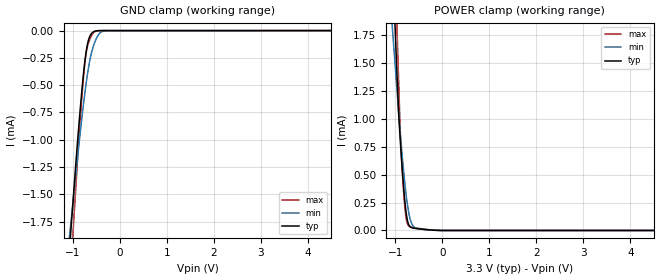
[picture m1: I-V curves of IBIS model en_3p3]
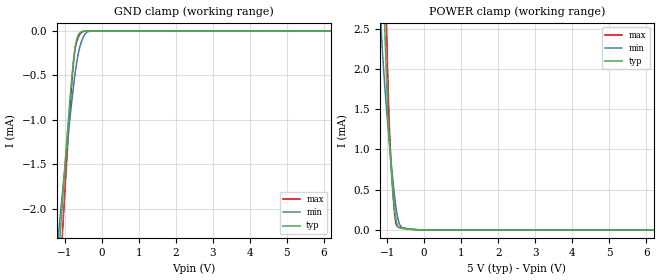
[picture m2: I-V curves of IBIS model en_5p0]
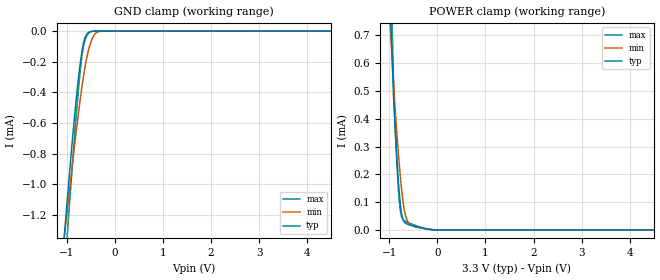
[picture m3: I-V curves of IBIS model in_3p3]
|Texas Instruments Incorporated
| ISO734x Robust EMC, Low Power, Quad-Channel Digital Isolators
| Marketing part#   Digital Voltage Range   Package-type   #pins
| ISO7341CDW   3.0V - 5.5V   SOIC   16
[IBIS Ver]   4.1
[File name]   iso7341c.ibs
[File Rev]   1.1
[Date]   9/10/2014
[Source]
| Texas Instruments Incorporated.
| Analog-eLab Design Center, HPA
| 12500 TI Blvd
| Dallas, TX -75243
[Notes]   Revision History:
| Rev 1.1: 9/10/2014
| - output_3p3 and output_5p0 modeled as tri-state buffers.
| Rev 1.0: 8/19/2014
| - Initial version of the model.
| - Model generated from simulations in SPECTRE
| - Model matched to SPICE simulation
| - C_comp although listed in numerical order of value are
|   obtained from varying PVT conditions. For PVT conditions for
|   each specific value refer the buffer description under
|   respective [Model]. IBIS model user is responsible for using
|   appropriate C_comp to simulate for Signal Integrity.
| - Model names with a trailing _3p3 contains the model for
|   3.3V [3.0V and 3.6V]. Model names with a trailing _5p0 contains
|   the model for 5V [4.5V and 5.5V].
| - GND Clamp non monotonic for EN and IN input buffers.
| - IBIS model created from existing model of ISO7342.
[Disclaimer]
| This model is designed as an aid for customers of Texas Instruments.
| TI and its licensors and suppliers make no warranties, either expressed
| or implied, with respect to this  model, including the warranties of
| merchantability or fitness for a particular purpose. The model is
| provided solely on an "as is" basis. The entire risk as to its quality
| and performance is with the customer.
[Copyright]
(C) Copyright 2014 Texas Instruments Incorporated.All rights reserved.
|   ISO7341CDW
[Component]   ISO7341CDW
[Manufacturer]   TI
[Package]   |16 SOIC  -  DW package
|   typ   min   max
R_pkg   0.13983   0.12494   0.1793
L_pkg   2.1802nH   1.9245nH   2.8571nH
C_pkg   0.42060pF   0.2145pF   0.61276pF
[Pin]   signal_name   model_name   R_pin   L_pin   C_pin
1   VCC1   POWER   0.09703  2.25823nH  0.63889pF
2   GND1   GND   0.10567  2.15194nH  0.30706pF
3   INA   IN   0.12889  1.99554nH  0.21450pF
4   INB   IN   0.12623  1.94755nH  0.61276pF
5   INC   IN   0.12494  1.92646nH  0.36666pF
6   OUTD   OUT   0.14038  2.18765nH  0.43235pF
7   EN1   EN   0.17807  2.83638nH  0.45904pF
8   GND1   GND   0.08216  2.43955nH  0.44498pF
9   GND2   GND   0.10126  2.44074nH  0.40934pF
10   EN2   EN   0.17928  2.85707nH  0.52717pF
11   IND   IN   0.12883  1.99615nH  0.50841pF
12   OUTC   OUT   0.12617  1.94399nH  0.32633pF
13   OUTB   OUT   0.12498  1.92454nH  0.37783pF
14   OUTA   OUT   0.14050  2.18615nH  0.38097pF
15   GND2   GND   0.08275  2.09014nH  0.75096pF
16   VCC2   POWER   0.09747  2.26909nH  0.67439pF
|   Model Selectors
[Model Selector] EN
en_3p3   3.3V digital Input
en_5p0   5.0V digital Input
[Model Selector] IN
in_3p3   3.3V digital Input
in_5p0   5.0V digital Input
[Model Selector] OUT
output_3p3   3.3V digital 3-state
output_5p0   5.0V digital 3-state
| Models and submodels in the file (6): en_3p3 (Input), en_5p0 (Input), in_3p3 (Input), in_5p0 (Input), output_3p3 (3-state), output_5p0 (3-state)
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|   en_3p3 Model
[Model]   en_3p3
Model_type   Input
Vinl = 0.8
Vinh = 2
|   typ   min   max
|   (nom PVT)   (slow PVT)   (fast PVT)
C_comp   0.161pF   0.098pF   0.252pF
| Where   nom PVT is  Nominal Process, 3.3V, 27C
|   Fast PVT is Strong Process, 3.6V, -40C
|   Slow PVT is Weak Process, 3.0V, 150C
[Voltage Range]   3.3   3   3.6
[Temperature Range]   27   150   -40
[Power Clamp Reference]   3.3   3   3.6
[GND Clamp Reference]   0   0   0
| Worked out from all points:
|   GND clamp passes 1 mA (typ) near -0.90 V on its own axis
|   POWER clamp passes 1 mA (typ) near -0.92 V on its own axis
[GND Clamp]
|   Voltage   I(typ)   I(min)   I(max)
-3.3V     -16.02mA   -12.12mA   -20.07mA
-1.082V   -2.058mA   -1.927mA   -2.435mA
-933.9mV  -1.195mA   -1.301mA   -1.409mA
-815.1mV  -576.9uA   -823.1uA   -642.6uA
-775.5mV  -399.7uA   -677.1uA   -429.5uA
-735.9mV  -249.5uA   -540.6uA   -261.7uA
-696.3mV  -138.4uA   -417.2uA   -157.1uA
-656.7mV  -70.87uA   -311.6uA   -97.71uA
-547.8mV  -8.269uA   -122.2uA   -15.56uA
-438.9mV  -609.9nA   -28.59uA   -715.7nA
-300.3mV  -135.4nA   -1.693uA   -73.15nA
6.6V      0A         0A         0A
[POWER Clamp]
|   Voltage   I(typ)   I(min)   I(max)
-3.3V     37.87mA    27.97mA    46.61mA
-1.082V   2.59mA     1.912mA    3.362mA
-933.9mV  1.066mA    1.077mA    1.378mA
-894.3mV  792.6uA    854.2uA    848.9uA
-844.8mV  490.1uA    618.8uA    468.6uA
-795.3mV  245.9uA    408.6uA    190uA
-765.6mV  141.6uA    299.7uA    94.29uA
-735.9mV  76.12uA    208uA      52.02uA
-656.7mV  25.39uA    64.33uA    30.38uA
-518.1mV  15.3uA     15.27uA    20.19uA
-3.3mV    22.97nA    56.83nA    14.08nA
6.6V      0A         0A         0A
|   en_5p0 Model
[Model]   en_5p0
Model_type   Input
Vinl = 0.8
Vinh = 2
|   typ   min   max
|   (nom PVT)   (slow PVT)   (fast PVT)
C_comp   0.173pF   0.101pF   0.247pF
| Where   nom PVT is  Nominal Process, 5.0V, 27C
|   Fast PVT is Strong Process, 5.5V, -40C
|   Slow PVT is Weak Process, 4.5V, 150C
[Voltage Range]   5   4.5   5.5
[Temperature Range]   27   150   -40
[Power Clamp Reference]   5   4.5   5.5
[GND Clamp Reference]   0   0   0
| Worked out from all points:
|   GND clamp passes 1 mA (typ) near -0.90 V on its own axis
|   POWER clamp passes 1 mA (typ) near -0.92 V on its own axis
[GND Clamp]
|   Voltage   I(typ)   I(min)   I(max)
-5V       -26.85mA   -20.05mA   -33.83mA
-1.235V   -2.983mA   -2.6mA     -3.546mA
-1.13V    -2.354mA   -2.134mA   -2.795mA
-1.115V   -2.264mA   -2.068mA   -2.688mA
-1.055V   -1.904mA   -1.808mA   -2.259mA
-860mV    -799.2uA   -997uA     -914.7uA
-755mV    -317.8uA   -605uA     -335.4uA
-665mV    -81.82uA   -332uA     -109.5uA
-530mV    -5.449uA   -101.8uA   -10.68uA
-425mV    -437.8nA   -22.05uA   -447nA
-275mV    -117.8nA   -1.166uA   -60.6nA
10V       0A         0A         0A
[POWER Clamp]
|   Voltage   I(typ)   I(min)   I(max)
-5V       66.01mA    49.38mA    80.54mA
-1.235V   4.734mA    3.205mA    6.08mA
-1.13V    3.373mA    2.244mA    4.359mA
-1.085V   2.789mA    1.93mA     3.621mA
-1.055V   2.4mA      1.739mA    3.129mA
-1.025V   2.011mA    1.559mA    2.638mA
-980mV    1.427mA    1.304mA    1.9mA
-935mV    1.075mA    1.063mA    1.241mA
-845mV    491.9uA    621.1uA    470.4uA
-770mV    155.2uA    316.2uA    105.1uA
-650mV    24.69uA    59.36uA    30.24uA
10V       0A         0A         0A
|   in_3p3 Model
[Model]   in_3p3
Model_type   Input
Vinl = 0.8
Vinh = 2
|   typ   min   max
|   (nom PVT)   (slow PVT)   (fast PVT)
C_comp   0.351pF   0.323pF   0.382pF
| Where   nom PVT is  Nominal Process, 3.3V, 27C
|   Fast PVT is Strong Process, 3.6V, -40C
|   Slow PVT is Weak Process, 3.0V, 150C
[Voltage Range]   3.3   3   3.6
[Temperature Range]   27   150   -40
[Power Clamp Reference]   3.3   3   3.6
[GND Clamp Reference]   0   0   0
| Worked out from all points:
|   GND clamp passes 1 mA (typ) near -0.96 V on its own axis
|   POWER clamp passes 1 mA (typ) near -1.02 V on its own axis
[GND Clamp]
|   Voltage   I(typ)   I(min)   I(max)
-3.3V     -10.5mA    -8.177mA   -12.99mA
-1.082V   -1.445mA   -1.431mA   -1.727mA
-914.1mV  -816.9uA   -954.1uA   -998.5uA
-805.2mV  -448.8uA   -657.2uA   -556.2uA
-716.1mV  -199.7uA   -434.2uA   -244.8uA
-676.5mV  -117.1uA   -344.3uA   -142.2uA
-636.9mV  -59.87uA   -263.2uA   -75.98uA
-587.4mV  -22.32uA   -177.9uA   -31.66uA
-528mV    -5.765uA   -100.5uA   -8.109uA
-419.1mV  -436.4nA   -19.72uA   -339.2nA
-260.7mV  -145.3nA   -1.051uA   -79.88nA
6.6V      0A         0A         0A
[POWER Clamp]
|   Voltage   I(typ)   I(min)   I(max)
-3.3V     19.35mA    14.36mA    23.78mA
-1.082V   1.282mA    1.032mA    1.702mA
-914.1mV  486.5uA    539.1uA    550.7uA
-894.3mV  418uA      481uA      439.2uA
-844.8mV  262.9uA    353.4uA    248.9uA
-805.2mV  160.1uA    262.6uA    132.8uA
-775.5mV  100.8uA    201.4uA    76.11uA
-706.2mV  34.28uA    91.86uA    35.49uA
-627mV    21.23uA    34.25uA    27.78uA
-488.4mV  13.81uA    12.6uA     18.19uA
-3.3mV    4.025nA    17.39nA    2.182nA
6.6V      0A         0A         0A
